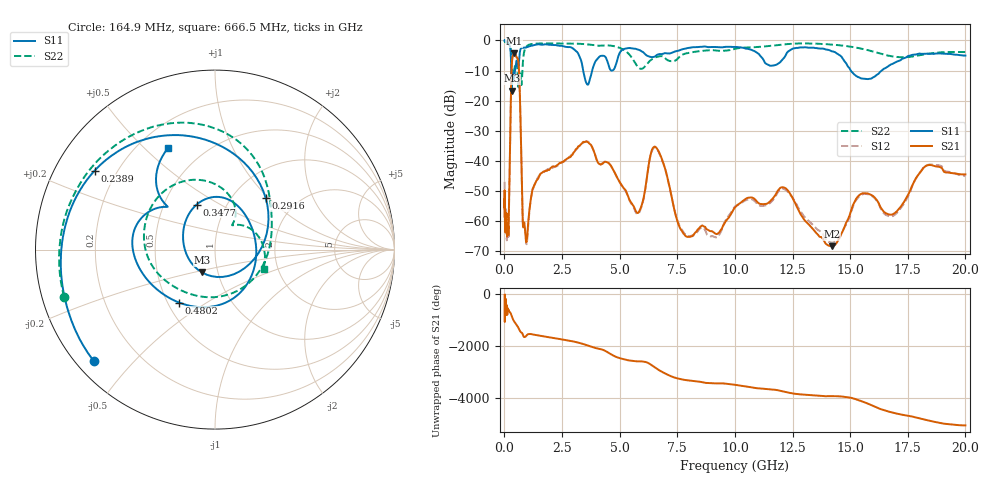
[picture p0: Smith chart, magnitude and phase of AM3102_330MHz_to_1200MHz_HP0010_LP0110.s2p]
! Date/Time: Tue, Sep 11, 2018 5:10 PM
! Network Analyzer: Agilent Technologies E8362B Rev: A.07.50.63
! Sweep from 0.010 to 20.000 GHz, 1601 Points, Sweep Type: LOG
! Power Supply: 4.950 V, 0.001 A
# Hz S DB R 50
!freq MagS11 AngS11 MagS21 AngS21 MagS12 AngS12 MagS22 AngS22
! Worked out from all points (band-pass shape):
!   1601 points, 10 MHz to 20 GHz, reference 50 ohm
!   highest |S21| = -4.26 dB at 420.4 MHz (marker M1); lowest = -68.4 dB at 14.21 GHz (marker M2)
!   |S21| within 3 dB of the highest: 326.8 MHz to 608.2 MHz (281.4 MHz wide, 60.2 % of centre)
!   lowest |S11| = -16.7 dB at 319.2 MHz (marker M3), VSWR 1.34, Z = 42 - j10.9 ohm
!   |S11| at or under -10 dB: 297.6 MHz to 460.4 MHz (162.7 MHz wide, 42.9 % of centre); 3.417 GHz to 3.808 GHz (390.5 MHz wide, 10.8 % of centre); 15.03 GHz to 16.37 GHz (1.344 GHz wide, 8.56 % of centre)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
!   |S22| runs from -15.6 to -0.2 dB; largest |S21 - S12| = 0.01
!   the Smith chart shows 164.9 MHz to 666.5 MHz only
!   S11 on the Smith chart (normalised r, x): 164.9 MHz: 0.05, -0.39; 238.9 MHz: 0.12, +0.29; 291.6 MHz: 1.40, +0.96; 347.7 MHz: 0.72, +0.39; 480.2 MHz: 0.57, -0.39; 666.5 MHz: 0.32, +0.59
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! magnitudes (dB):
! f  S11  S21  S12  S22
! 10 MHz  0.0  -55.3  -47.0  -0.2
! 35.55 MHz  0.0  -60.4  -60.1  -0.4
! 126.4 MHz  -0.4  -62.6  -62.7  -0.9
! 164.9 MHz  -0.7  -62.1  -65.6  -1.1
! 238.9 MHz  -1.9  -38.5  -38.7  -1.8
! 291.6 MHz  -7.9  -15.5  -15.5  -3.9
! 319.2 MHz  -16.7  -8.3  -8.3  -7.4
! 347.7 MHz  -11.4  -5.7  -5.8  -10.5
! 420.4 MHz  -12.5  -4.3  -4.3  -10.0
! 447.2 MHz  -10.7  -4.4  -4.4  -8.7
! 480.2 MHz  -9.0  -4.7  -4.8  -7.7
! 666.5 MHz  -4.1  -16.6  -16.7  -10.7
! 794.6 MHz  -2.5  -59.6  -60.3  -8.3
! 951.8 MHz  -2.3  -66.7  -67.7  -2.0
! 1.59 GHz  -1.4  -44.2  -44.3  -1.0
! 3.599 GHz  -14.6  -33.7  -33.6  -1.3
! 5.652 GHz  -2.7  -55.9  -56.3  -7.2
! 6.58 GHz  -5.0  -35.6  -35.8  -5.5
! 7.882 GHz  -2.7  -65.1  -64.6  -4.3
! 12.09 GHz  -6.2  -48.8  -49.3  -1.3
! 14.21 GHz  -3.6  -68.4  -67.3  -1.4
! 20 GHz  -5.0  -44.5  -45.2  -3.9
